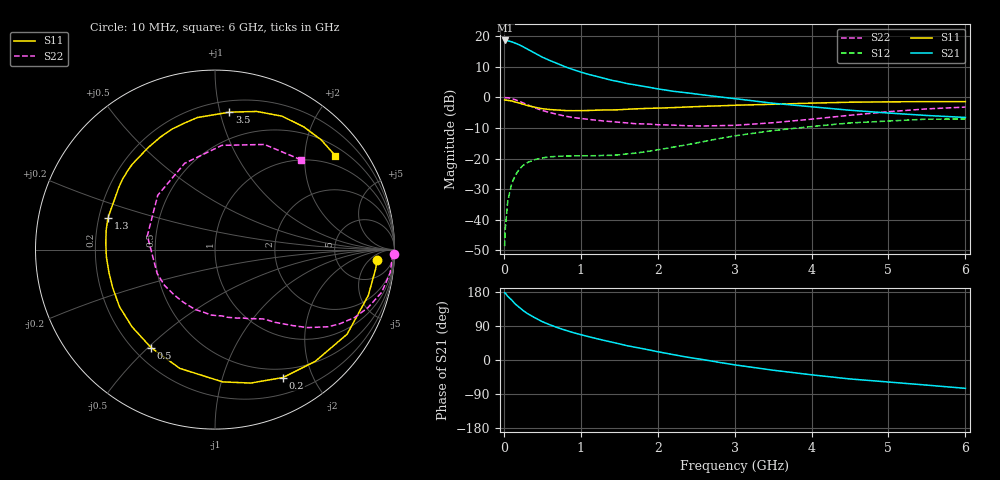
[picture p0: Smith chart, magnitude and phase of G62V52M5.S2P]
! SIEMENS Small Signal Semiconductors
! BFG193
! Si NPN RF Bipolar Junction Transistor in SOT223
! VCE = 2.5 V  IC = 2.5 mA
! Common Emitter S-Parameters:  August  1996
# GHz  S  MA  R  50
!  f  S11  S21  S12  S22
! GHz  MAG  ANG  MAG  ANG  MAG  ANG  MAG  ANG
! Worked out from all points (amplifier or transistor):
!   36 points, 10 MHz to 6 GHz, reference 50 ohm
!   highest |S21| = 18.6 dB at 20 MHz (marker M1)
!   |S21| within 3 dB of that: start of sweep to 319.6 MHz
!   unconditionally stable (mu >= 1): 1.321 GHz to 2.612 GHz
!   at 250 MHz: K = 0.21, MSG = 19.4 dB, |S12| = -22.2 dB
!   at 1.4 GHz: K = 1.07, MAG = 10.7 dB, |S12| = -19.0 dB
!   at 6 GHz: K = 0.95, MSG = 0.3 dB, |S12| = -7.1 dB
!   S11 on the Smith chart (normalised r, x): 10 MHz: 15, -9; 200 MHz: 0.39, -1.60; 500 MHz: 0.27, -0.51; 1.3 GHz: 0.24, +0.14; 3.5 GHz: 0.28, +1.07; 6 GHz: 0.73, +2.74
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0.01  0.906 -3.5  8.434 177.6  0.0037 91.4  0.9959 -1.5
0.02  0.9015 -6.8  8.496 176.2  0.0074 88.3  0.9877 -2.9
0.05  0.8916 -16.6  8.403 168.1  0.0197 80.3  0.9848 -7.5
0.1  0.8741 -32.6  8.093 158.7  0.0381 73.1  0.9587 -14.4
0.15  0.8365 -48.0  7.663 147.4  0.0537 63.8  0.9113 -20.8
0.2  0.8072 -62.0  7.206 139.1  0.0667 57.6  0.8644 -26.0
0.25  0.7698 -75.0  6.705 130.7  0.0772 51.1  0.8091 -30.7
0.3  0.7382 -86.7  6.201 123.4  0.0853 46.5  0.7629 -34.3
0.4  0.6903 -106.5  5.306 111.8  0.0958 38.1  0.6747 -40.1
0.5  0.6522 -123.1  4.528 101.2  0.1023 32.0  0.6093 -44.1
0.6  0.6314 -137.1  3.991 92.8  0.1069 28.3  0.5634 -47.3
0.7  0.62 -149.1  3.546 85.3  0.1087 25.5  0.525 -50.5
0.9  0.6045 -168.1  2.842 72.4  0.1106 22.5  0.4683 -55.5
1.1  0.6095 176.6  2.376 61.7  0.1111 21.7  0.4361 -61.9
1.3  0.6219 163.6  2.051 51.9  0.1125 22.6  0.4103 -68.1
1.6  0.638 147.3  1.681 37.8  0.119 25.7  0.3825 -80.0
2.2  0.6794 123.2  1.257 14.3  0.1533 30.2  0.3514 -108.5
2.8  0.7257 103.3  1.018 -6.3  0.2118 26.0  0.3447 -144.7
3.5  0.77 84.0  0.8 -26.9  0.2863 11.9  0.3847 168.5
4.5  0.832 63.3  0.615 -50.0  0.3818 -10.8  0.5095 109.4
5.5  0.8509 46.0  0.505 -66.3  0.4401 -38.3  0.6474 64.8
6  0.8503 37.9  0.469 -74.8  0.4422 -53.3  0.6929 46.2
